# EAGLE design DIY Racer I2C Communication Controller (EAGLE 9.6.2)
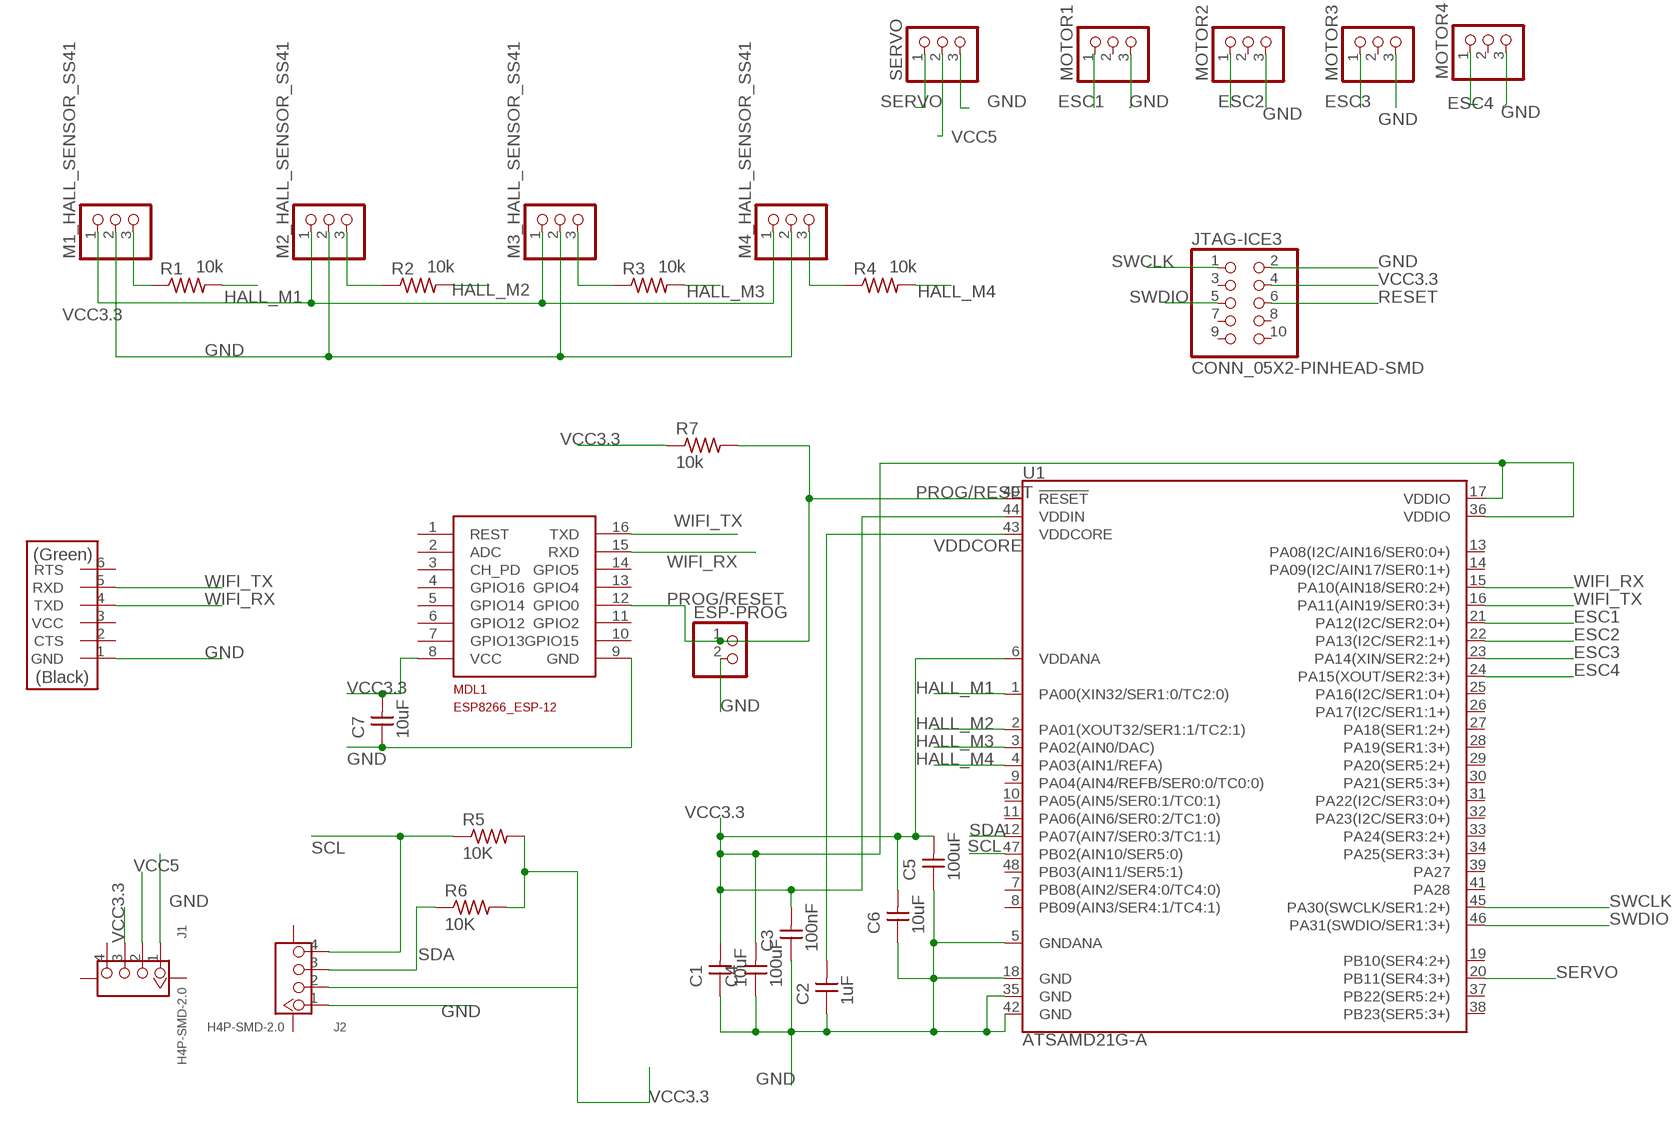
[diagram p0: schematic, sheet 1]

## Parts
C1  10uF  CAP_UNPOLARIZED  [C1206]
C2  1uF  CAP_UNPOLARIZED  [C1206]
C3  100nF  CAP_UNPOLARIZED  [C1206]
C4  100uF  CAP_UNPOLARIZED  [C1206]
C5  100uF  CAP_UNPOLARIZED  [C1206]
C6  10uF  CAP_UNPOLARIZED  [C1206]
C7  10uF  CAP_UNPOLARIZED  [C1206]
ESP-PROG  PINHD-1X02_2.54-SMD  [1X02SMD]
FTDI  CONN_06_FTDI-SMD-HEADER  [1X06SMD]
J1  H4P-SMD-2.0  GROVE-CONNECTOR-SMD(4+2P-2.0)  [HW4-SMD-2.0]
J2  H4P-SMD-2.0  GROVE-CONNECTOR-SMD(4+2P-2.0)  [HW4-SMD-2.0]
JTAG-ICE3  CONN_05X2-PINHEAD-SMD  [2X05SMD]
M1_HALL_SENSOR_SS41  PINHD-1X03_2.54-SMD  [1X03SMD]
M2_HALL_SENSOR_SS41  PINHD-1X03_2.54-SMD  [1X03SMD]
M3_HALL_SENSOR_SS41  PINHD-1X03_2.54-SMD  [1X03SMD]
M4_HALL_SENSOR_SS41  PINHD-1X03_2.54-SMD  [1X03SMD]
MDL1  ESP8266-12GPIO04/05_CORRECTED  [ESP8266-ESP12]
MOTOR1  PINHD-1X03_2.54-SMD  [1X03SMD]
MOTOR2  PINHD-1X03_2.54-SMD  [1X03SMD]
MOTOR3  PINHD-1X03_2.54-SMD  [1X03SMD]
MOTOR4  PINHD-1X03_2.54-SMD  [1X03SMD]
R1  10k  R1206FAB  [R1206FAB]
R2  10k  R1206FAB  [R1206FAB]
R3  10k  R1206FAB  [R1206FAB]
R4  10k  R1206FAB  [R1206FAB]
R5  10K  R1206FAB  [R1206FAB]
R6  10K  R1206FAB  [R1206FAB]
R7  10k  R1206FAB  [R1206FAB]
SERVO  PINHD-1X03_2.54-SMD  [1X03SMD]
U1  ATSAMD21G-A  [TQFP-48]

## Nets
ESC1: MOTOR1.1 U1.21(PA12(I2C/SER2:0+))
ESC2: MOTOR2.1 U1.22(PA13(I2C/SER2:1+))
ESC3: MOTOR3.1 U1.23(PA14(XIN/SER2:2+))
ESC4: MOTOR4.1 U1.24(PA15(XOUT/SER2:3+))
GND: C1.1 C2.1 C3.1 C4.1 C5.1 C6.1 C7.1 ESP-PROG.2 FTDI.1(GND) J1.1 J2.1 JTAG-ICE3.2 M1_HALL_SENSOR_SS41.2 M2_HALL_SENSOR_SS41.2 M3_HALL_SENSOR_SS41.2 M4_HALL_SENSOR_SS41.2 MDL1.9(GND) MOTOR1.3 MOTOR2.3 MOTOR3.3 MOTOR4.3 SERVO.3 U1.5(GNDANA) U1.18(GND) U1.35(GND) U1.42(GND)
HALL_M1: R1.2 U1.1(PA00(XIN32/SER1:0/TC2:0))
HALL_M2: R2.2 U1.2(PA01(XOUT32/SER1:1/TC2:1))
HALL_M3: R3.2 U1.3(PA02(AIN0/DAC))
HALL_M4: R4.2 U1.4(PA03(AIN1/REFA))
N$1: M1_HALL_SENSOR_SS41.3 R1.1
N$2: M2_HALL_SENSOR_SS41.3 R2.1
N$3: M3_HALL_SENSOR_SS41.3 R3.1
N$4: M4_HALL_SENSOR_SS41.3 R4.1
PROG/RESET: ESP-PROG.1 MDL1.12(GPIO0) R7.2 U1.40(!RESET!)
RESET: JTAG-ICE3.6
SCL: J2.4 R5.1 U1.47(PB02(AIN10/SER5:0))
SDA: J2.3 R6.1 U1.12(PA07(AIN7/SER0:3/TC1:1))
SERVO: SERVO.1 U1.20(PB11(SER4:3+))
SWCLK: JTAG-ICE3.1 U1.45(PA30(SWCLK/SER1:2+))
SWDIO: JTAG-ICE3.5 U1.46(PA31(SWDIO/SER1:3+))
VCC3.3: C1.2 C3.2 C4.2 C5.2 C6.2 C7.2 J1.3 J2.2 JTAG-ICE3.4 M1_HALL_SENSOR_SS41.1 M2_HALL_SENSOR_SS41.1 M3_HALL_SENSOR_SS41.1 M4_HALL_SENSOR_SS41.1 MDL1.8(VCC) R5.2 R6.2 R7.1 U1.6(VDDANA) U1.17(VDDIO) U1.36(VDDIO) U1.44(VDDIN)
VCC5: J1.2 SERVO.2
VDDCORE: C2.2 U1.43(VDDCORE)
WIFI_RX: FTDI.4(TXD) MDL1.15(RXD) U1.15(PA10(AIN18/SER0:2+))
WIFI_TX: FTDI.5(RXD) MDL1.16(TXD) U1.16(PA11(AIN19/SER0:3+))
Unconnected: FTDI.2(CTS) FTDI.3(VCC) FTDI.6(RTS) J1.4 J1.SS1 J1.SS2 J2.SS1 J2.SS2 JTAG-ICE3.3 JTAG-ICE3.7 JTAG-ICE3.8 JTAG-ICE3.9 JTAG-ICE3.10 MDL1.1(REST) MDL1.2(ADC) MDL1.3(CH_PD) MDL1.4(GPIO16) MDL1.5(GPIO14) MDL1.6(GPIO12) MDL1.7(GPIO13) MDL1.10(GPIO15) MDL1.11(GPIO2) MDL1.13(GPIO4) MDL1.14(GPIO5) MOTOR1.2 MOTOR2.2 MOTOR3.2 MOTOR4.2 U1.7(PB08(AIN2/SER4:0/TC4:0)) U1.8(PB09(AIN3/SER4:1/TC4:1)) U1.9(PA04(AIN4/REFB/SER0:0/TC0:0)) U1.10(PA05(AIN5/SER0:1/TC0:1)) U1.11(PA06(AIN6/SER0:2/TC1:0)) U1.13(PA08(I2C/AIN16/SER0:0+)) U1.14(PA09(I2C/AIN17/SER0:1+)) U1.19(PB10(SER4:2+)) U1.25(PA16(I2C/SER1:0+)) U1.26(PA17(I2C/SER1:1+)) U1.27(PA18(SER1:2+)) U1.28(PA19(SER1:3+)) U1.29(PA20(SER5:2+)) U1.30(PA21(SER5:3+)) U1.31(PA22(I2C/SER3:0+)) U1.32(PA23(I2C/SER3:0+)) U1.33(PA24(SER3:2+)) U1.34(PA25(SER3:3+)) U1.37(PB22(SER5:2+)) U1.38(PB23(SER5:3+)) U1.39(PA27) U1.41(PA28) U1.48(PB03(AIN11/SER5:1))

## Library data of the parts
C1-C7 = fab:CAP_UNPOLARIZED
ESP-PROG = pinhead-2:PINHD-1X02: PIN HEADER
FTDI = fab:CONN_06_FTDI-SMD-HEADER
J1 J2 = OPL_Connector:GROVE-CONNECTOR-SMD(4+2P-2.0): 320110030
JTAG-ICE3 = fab:CONN_05X2-PINHEAD-SMD
M1_HALL_SENSOR_SS41 M2_HALL_SENSOR_SS41 M3_HALL_SENSOR_SS41 M4_HALL_SENSOR_SS41 MOTOR1-MOTOR4 SERVO = pinhead-2:PINHD-1X03: PIN HEADER
MDL1 = ESP8266-ESP12:ESP8266-12: Espressif ESP8266 ESP-12 Module with GPIO04 and GPIO05 corrected.
R1-R7 = fab:R: Resistor (US Symbol)
U1 = samd21-temp:ATSAMD21G: Atmel SAMD21G SMART ARM-Based Microcontroller The Atmel ® | SMART ™ SAM D21 is a series of low-power microcontrollers using the 32-bit ARM ® Cortex ® -M0+ processor, and ranging from 32- to 64-pins with up to 256KB Flash and 32KB of SRAM. The SAM D21 devices operate at a maximum frequency of 48MHz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; PROD_ID: IC-13064

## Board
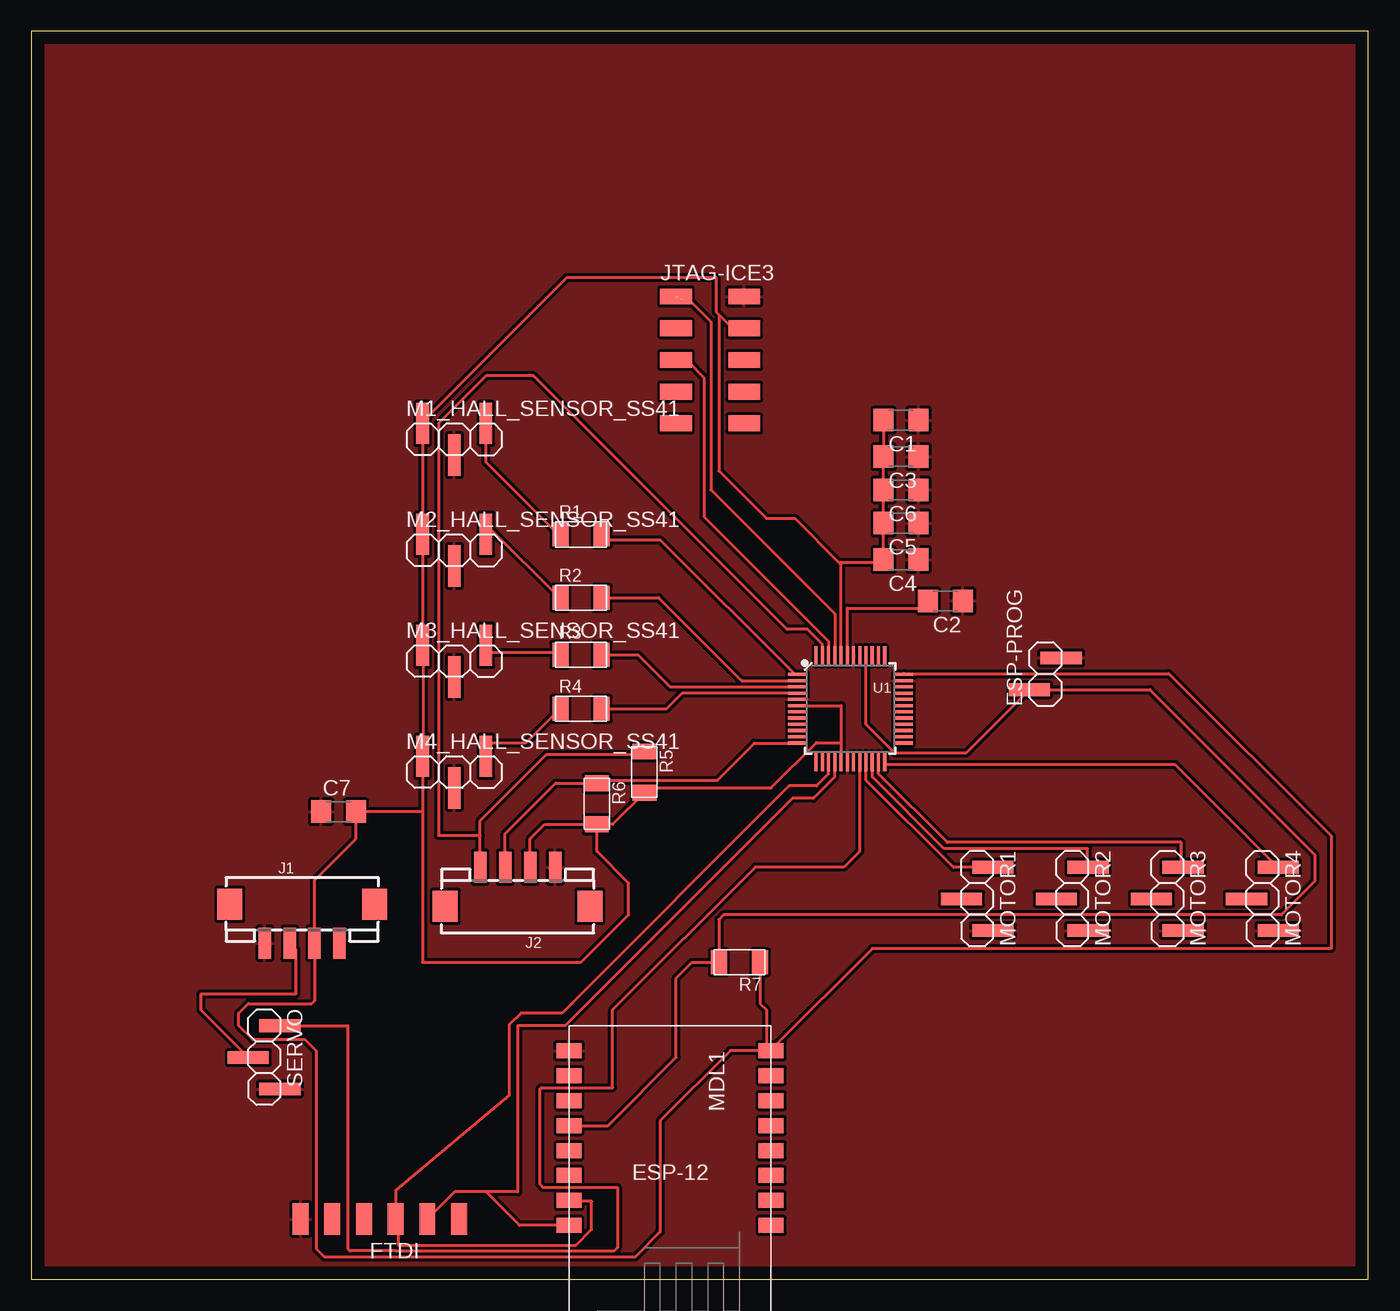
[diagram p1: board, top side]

Size 107.17 x 100 mm. Coordinates in mm from the lower left corner, seen from the top.
Outline: 0,0 107.17,0 107.17,100 0,100 0,0
Copper layers (1*16): Top 0.035mm / dielectric 1.5mm / Bottom 0.035mm
Design rules "default *": minimum track width 0.24mm, minimum drill 0.35mm, track to track 0.25mm, track to pad 0.23mm, pad to pad 0.23mm, via to via 0.4mm, smd to smd 0.23mm, copper to edge 40mil, drill to drill 6mil, minimum pad ring 10mil, minimum via ring 8mil, stop-mask expansion 4mil, vias tented up to drill 0mil, thermal gap 10mil

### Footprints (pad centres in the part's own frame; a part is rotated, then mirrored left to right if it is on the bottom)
C1206 = smd 1.6 x 1.8: 1 -1.4,0; 2 1.4,0
1X02SMD = smd 1.016 x 3.302: 1 -1.27,1.27; 2 1.27,-1.27
1X06SMD = smd 2.54 x 1.27: 1 0,6.35; 2 0,3.81; 3 0,1.27; 4 0,-1.27; 5 0,-3.81; 6 0,-6.35
HW4-SMD-2.0 = smd 1 x 2.5: 1 -3,0; 2 -1,0; 3 1,0; 4 3,0 | smd 2 x 2.5: SS1 -5.8,3.123; SS2 5.8,3.123
2X05SMD = smd 2.54 x 1.27: 1 -2.54,2.54; 2 2.92,2.54; 3 -2.54,0; 4 2.92,0; 5 -2.54,-2.54; 6 2.92,-2.54; 7 -2.54,-5.08; 8 2.92,-5.08; 9 -2.54,-7.62; 10 2.92,-7.62
1X03SMD = smd 1.016 x 3.302: 1 -1.27,1.27; 2 1.27,-1.27; 3 3.81,1.27
ESP8266-ESP12 = smd 2 x 1.2: 1 0,16; 2 0,14; 3 0,12; 4 0,10; 5 0,8; 6 0,6; 7 0,4; 8 0,2; 9 16.2,2; 10 16.2,4; 11 16.2,6; 12 16.2,8; 13 16.2,10; 14 16.2,12; 15 16.2,14; 16 16.2,16
R1206FAB = smd 1.27 x 1.905: 1 -1.651,0; 2 1.651,0
TQFP-48 = smd 1.5 x 0.25: 1 -4.25,2.75; 2 -4.25,2.25; 3 -4.25,1.75; 4 -4.25,1.25; 5 -4.25,0.75; 6 -4.25,0.25; 7 -4.25,-0.25; 8 -4.25,-0.75; 9 -4.25,-1.25; 10 -4.25,-1.75; 11 -4.25,-2.25; 12 -4.25,-2.75; 25 4.25,-2.75; 26 4.25,-2.25; 27 4.25,-1.75; 28 4.25,-1.25; 29 4.25,-0.75; 30 4.25,-0.25; 31 4.25,0.25; 32 4.25,0.75; 33 4.25,1.25; 34 4.25,1.75; 35 4.25,2.25; 36 4.25,2.75 | smd 0.25 x 1.5: 13 -2.75,-4.25; 14 -2.25,-4.25; 15 -1.75,-4.25; 16 -1.25,-4.25; 17 -0.75,-4.25; 18 -0.25,-4.25; 19 0.25,-4.25; 20 0.75,-4.25; 21 1.25,-4.25; 22 1.75,-4.25; 23 2.25,-4.25; 24 2.75,-4.25; 37 2.75,4.25; 38 2.25,4.25; 39 1.75,4.25; 40 1.25,4.25; 41 0.75,4.25; 42 0.25,4.25; 43 -0.25,4.25; 44 -0.75,4.25; 45 -1.25,4.25; 46 -1.75,4.25; 47 -2.25,4.25; 48 -2.75,4.25

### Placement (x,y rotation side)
C1  69.72,68.83 180 top
C2  73.28,54.36 180 top
C3  69.72,65.91 180 top
C4  69.72,57.66 180 top
C5  69.72,60.58 180 top
C6  69.72,63.25 180 top
C7  24.64,37.47 0 top
ESP-PROG  81.28,48.51 90 top
FTDI  27.94,4.83 90 top
J1  21.72,26.92 0 top
J2  38.99,33.02 180 top
JTAG-ICE3  54.23,76.2 0 top
M1_HALL_SENSOR_SS41  32.64,67.31 0 top
M2_HALL_SENSOR_SS41  32.64,58.42 0 top
M3_HALL_SENSOR_SS41  32.64,49.53 0 top
M4_HALL_SENSOR_SS41  32.64,40.64 0 top
MDL1  59.31,20.32 180 top
MOTOR1  75.82,31.75 270 top
MOTOR2  83.44,31.75 270 top
MOTOR3  91.06,31.75 270 top
MOTOR4  98.68,31.75 270 top
R1  44.07,59.69 0 top
R2  44.07,54.61 0 top
R3  44.07,50.04 0 top
R4  44.07,45.72 0 top
R5  49.15,40.64 270 top
R6  45.34,38.1 270 top
R7  56.77,25.4 180 top
SERVO  18.67,19.05 270 top
U1  65.66,45.72 0 top

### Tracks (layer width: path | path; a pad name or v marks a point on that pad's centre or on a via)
ESC1
  Top 0.24: U1.21 66.92,41.25 66.92,40 73.92,33 76.92,33 MOTOR1.1
ESC2
  Top 0.24: U1.22 67.42,41.25 67.42,40.25 73.17,34.5 84.67,34.5 84.67,33.25 MOTOR2.1
ESC3
  Top 0.24: U1.23 67.92,41.25 67.92,40.5 73.42,35 92.17,35 92.17,33.25 MOTOR3.1
ESC4
  Top 0.24: U1.24 68.42,41.25 91.67,41.25 99.92,33 MOTOR4.1
GND
  pour Top: 0.51,100.33 107.57,100.33 107.57,0 0.51,0
HALL_M1
  Top 0.24: U1.1 61.17,48.5 50.42,59.25 45.92,59.25 45.92,59.5 R1.2
HALL_M2
  Top 0.24: R2.2 50.29,54.61 56.93,47.97 U1.2
HALL_M3
  Top 0.24: R3.2 48.64,50.04 51.21,47.47 U1.3
HALL_M4
  Top 0.24: R4.2 50.93,45.72 52.19,46.98 U1.4
N$1
  Top 0.24: R1.1 42.17,59.75 36.42,65.5 36.42,68.5 M1_HALL_SENSOR_SS41.3
N$2
  Top 0.24: R2.1 42.17,54.75 36.92,60 36.67,60 36.67,59.75 M2_HALL_SENSOR_SS41.3
N$3
  Top 0.24: R3.1 42.17,50.25 36.67,50.25 36.67,50.75 M3_HALL_SENSOR_SS41.3
N$4
  Top 0.24: R4.1 42.17,45.5 39.67,43 36.67,43 36.67,42 M4_HALL_SENSOR_SS41.3
PROG/RESET
  Top 0.24: U1.40 66.92,49.75 66.92,44.46 69.22,42.16 74.93,42.16 ESP-PROG.1 89.66,47.24 102.87,34.04 102.87,31.88 100.2,29.21 55.5,29.21 55.12,28.83 R7.2 52.96,25.4 51.69,24.13 51.69,17.78 46.23,12.32 MDL1.12
SCL
  Top 0.24: U1.47 63.41,50.89 62.23,52.07 60.58,52.07 40.26,72.39 36.45,72.39 32.64,68.58 32.64,35.56 35.99,35.56 | J2.4 35.99,35.56 | 35.99,35.56 35.99,36.75 41.28,42.04 48.89,42.04 R5.1
SDA
  Top 0.24: U1.12 57.96,42.97 54.99,40.01 45.59,40.01 R6.1 42.04,39.75 37.99,35.7 J2.3
SERVO
  Top 0.24: U1.20 66.41,34.29 65.14,33.02 58.04,33.02 46.61,21.59 46.61,15.37 40.89,15.37 40.77,15.24 40.77,7.62 41.02,7.37 46.99,7.37 46.99,2.54 46.71,2.26 29.22,2.26 29.19,2.29 25.53,2.29 25.4,2.41 25.4,20.32 SERVO.1
SWCLK  (1 unrouted)
  Top 0.24: 52.2,78.49 52.7,78.49 54.48,76.71 54.48,63.25 64.41,53.32 U1.45
SWDIO
  Top 0.24: U1.46 63.92,50 63.92,51.12 53.92,61.12 53.92,72.25 52.67,73.5 51.92,73.5 JTAG-ICE3.5
VCC3.3
  Top 0.24: 64.92,43 64.92,45.97 64.91,45.97 U1.6 | 64.92,43 64.92,41.5 U1.17 | R6.2 46.61,36.45 R5.2 49.53,39.37 59.29,39.37 62.92,43 64.92,43 | U1.36 69.92,48.5 69.95,48.54 91.17,48.54 104.19,35.52 104.19,26.5 67.42,26.5 59.42,18.5 MDL1.8 58.93,18.32 | 55.12,77.3 56.17,76.25 56.92,76.25 JTAG-ICE3.4 | 55.12,77.3 54.92,77.5 54.92,80.25 42.92,80.25 31.42,68.75 M1_HALL_SENSOR_SS41.1 31.42,68.5 31.42,59.75 M2_HALL_SENSOR_SS41.1 31.42,59.5 31.42,51 M3_HALL_SENSOR_SS41.1 31.42,50.75 31.42,42 M4_HALL_SENSOR_SS41.1 31.37,37.47 | 55.12,77.3 55.12,64.77 58.93,60.96 61.21,60.96 64.71,57.47 | C1.2 C3.2 C6.2 C5.2 C4.2 68.32,57.4 68.26,57.47 64.71,57.47 | 31.37,37.47 31.37,25.4 44.07,25.4 47.88,29.21 47.88,31.75 45.34,34.29 R6.2 | R6.2 41.15,36.45 39.99,35.29 J2.2 | 64.71,57.47 64.91,57.27 U1.44 | 58.93,18.32 56.04,18.32 50.42,12.7 50.42,3.81 48.38,1.77 23.5,1.77 22.86,2.41 22.86,18.29 21.97,19.18 17.78,19.18 16.64,20.32 16.64,21.34 17.4,22.1 22.48,22.1 22.72,22.34 J1.3 22.72,31.99 26.04,35.31 26.04,36.83 | 26.04,36.83 C7.2 | 26.04,36.83 26.67,37.47 31.37,37.47 | R7.1 58.42,22.1 58.93,21.59 58.93,18.32
VCC5
  Top 0.24: J1.2 21.21,26.43 21.21,22.86 13.59,22.86 13.59,21.59 SERVO.2
VDDCORE
  Top 0.24: C2.2 71.3,53.78 65.41,53.78 U1.43
WIFI_RX
  Top 0.24: U1.15 63.92,41.25 63.92,40.5 62.95,39.53 60.74,39.53 42.55,21.34 39.24,21.34 38.31,20.4 38.31,14.73 29.21,7.15 FTDI.4 29.42,4.75 29.42,2.75 43.67,2.75 44.92,4 44.92,6.25 43.17,6.25 MDL1.15
WIFI_TX
  Top 0.24: U1.16 64.42,41.25 64.42,40.25 62.69,38.52 61,38.52 42.8,20.32 38.99,20.32 38.99,7 36.45,7 | 36.45,7 33.92,7 31.92,5 FTDI.5 | MDL1.16 39.13,4.32 36.45,7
